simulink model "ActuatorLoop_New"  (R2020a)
settings: Solver=FixedStepDiscrete  StartTime=0.0  StopTime=10.0  FixedStep=0.001  RelTol=1e-3  EnableMultiTasking=on
model workspace (MAT data in the model file):
  Ts : Simulink.Parameter (value not decoded)

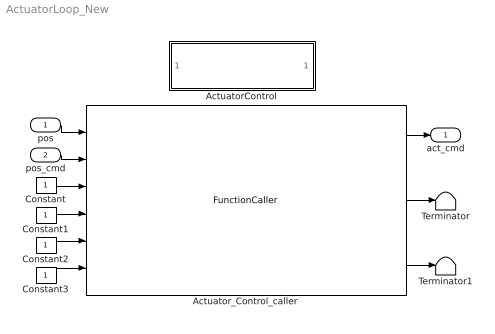
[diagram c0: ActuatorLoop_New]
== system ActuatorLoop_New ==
  pos : Inport  OutDataTypeStr=int16
  pos_cmd : Inport  Port=2  OutDataTypeStr=double
  ActuatorControl : ModelReference  ModelNameDialog=ActuatorControl.slx  SimulationMode=Normal  ScheduleRates=on  ModelReferenceVersion=1.70
  Actuator_Control_caller : FunctionCaller  FunctionPrototype=[Actuator1,Actuator2,Actuator3] = ActuatorControl.Actuator_Control(Act1_pos,Act1_cmd,Act2_pos,Act2_cmd,Act3_pos,Act3_cmd)  InputArgumentSpecifications=int16(1), double(1), int16(1), double(1), int16(1), double(1)  OutputArgumentSpecifications=int16(1), int16(1), int16(1)
  Constant : Constant  OutDataTypeStr=int16
  Constant1 : Constant  OutDataTypeStr=double
  Constant2 : Constant  OutDataTypeStr=int16
  Constant3 : Constant  OutDataTypeStr=double
  Terminator : Terminator
  Terminator1 : Terminator
  act_cmd : Outport
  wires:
  Constant/1 -> Actuator_Control_caller/3
  Actuator_Control_caller/2 -> Terminator/1
  Actuator_Control_caller/3 -> Terminator1/1
  Constant1/1 -> Actuator_Control_caller/4
  Constant2/1 -> Actuator_Control_caller/5
  Constant3/1 -> Actuator_Control_caller/6
  pos/1 -> Actuator_Control_caller/1
  pos_cmd/1 -> Actuator_Control_caller/2
  Actuator_Control_caller/1 -> act_cmd/1
